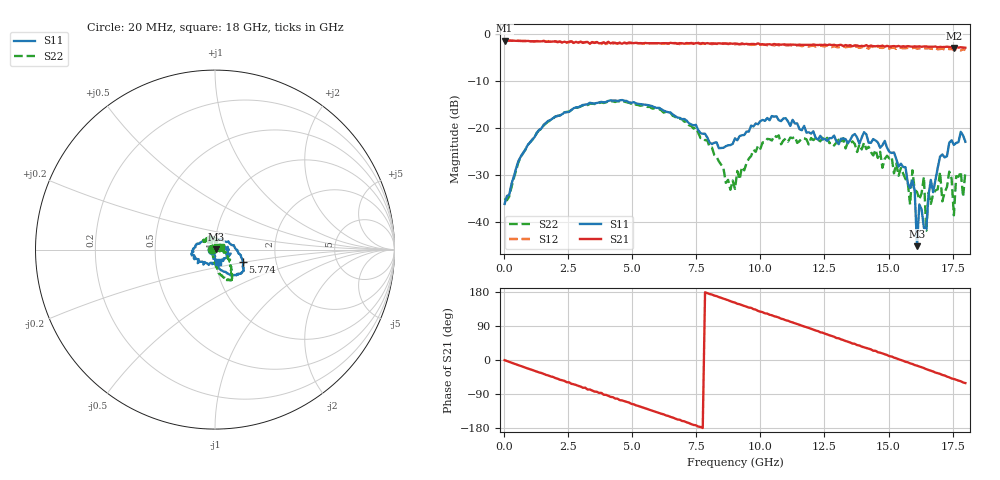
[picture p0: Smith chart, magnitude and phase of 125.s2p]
!Agilent Technologies,N5230A,US43500223,A.07.50.48
!Agilent N5230A: A.07.50.48
!Date: Tuesday, February 02, 2016 14:28:02
!Correction: S11(Full 2 Port(1,2))
!S21(Full 2 Port(1,2))
!S12(Full 2 Port(1,2))
!S22(Full 2 Port(1,2))
!S2P File: Measurements: S11, S21, S12, S22:
# Hz S  RI  R 50
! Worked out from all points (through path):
!   201 points, 20 MHz to 18 GHz, reference 50 ohm
!   highest |S21| = -1.32 dB at 20 MHz (marker M1); lowest = -2.9 dB at 17.55 GHz (marker M2)
!   group delay of S21, straight-line fit = 64.6 ps
!   lowest |S11| = -45.2 dB at 16.11 GHz (marker M3), VSWR 1.01, Z = 50.5 + j0.115 ohm
!   |S11| at or under -10 dB: start of sweep to end of sweep
!   |S22| runs from -41.9 to -14.3 dB; largest |S21 - S12| = 0.11
!   S11 on the Smith chart (normalised r, x): 20 MHz: 0.97, +0.00; 5.774 GHz: 1.36, -0.19; 18 GHz: 1.02, -0.14
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2e7  -0.0155 0.000255  0.8591 -0.00723  0.86 -0.0116  -0.0179 0.000888
1.2786e9  0.0115 -0.0887  0.7254 -0.4307  0.7272 -0.4344  0.00456 -0.0884
3.0766e9  0.103 -0.1431  0.2321 -0.7755  0.2216 -0.7891  0.0598 -0.1632
5.7736e9  0.1567 -0.0693  -0.5531 -0.584  -0.5767 -0.5584  0.0906 -0.1339
6.0433e9  0.155 -0.0555  -0.6129 -0.5207  -0.6336 -0.4911  0.0975 -0.1272
9.01e9  -0.0468 0.062  -0.7008 0.3827  -0.662 0.4162  0.00671 0.0214
1.02686e10  -0.1278 -0.00772  -0.4196 0.6598  -0.3502 0.6799  -0.062 0.0451
1.20666e10  -0.0351 -0.0852  0.1308 0.7681  0.1996 0.7354  -0.0365 0.0648
1.50333e10  0.0513 0.0218  0.7296 0.1297  0.7034 0.0536  -0.00156 0.0473
1.58424e10  0.00251 0.0228  0.7334 -0.1139  0.6833 -0.1878  -0.00134 0.0152
1.59323e10  0.012 0.0249  0.7256 -0.1336  0.6813 -0.2041  0.014 0.0325
1.61121e10  0.00538 0.00113  0.715 -0.1914  0.6533 -0.261  -0.00147 0.0208
1.6202e10  -0.0149 0.00336  0.7127 -0.2191  0.649 -0.2827  0.0107 0.0136
1.63818e10  0.00861 0.000151  0.6914 -0.2684  0.6226 -0.3435  0.028 0.0109
1.64717e10  0.0042 -0.00717  0.6784 -0.3048  0.6111 -0.3573  0.00713 0.00366
1.65616e10  -0.00609 -0.0181  0.6605 -0.325  0.5964 -0.3855  0.0124 0.0163
1.7101e10  -0.00866 -0.0516  0.5638 -0.4654  0.4828 -0.5115  0.0139 -0.00887
1.73707e10  0.0139 -0.0684  0.5107 -0.5246  0.4158 -0.5586  0.0333 0.00804
1.75505e10  0.00836 -0.0656  0.4594 -0.5488  0.3651 -0.5754  0.00979 0.00643
1.76404e10  0.0144 -0.0678  0.4501 -0.5783  0.3622 -0.592  0.0304 0.00384
1.79101e10  0.0195 -0.081  0.3693 -0.6218  0.2851 -0.6344  0.0184 -0.00111
1.8e10  0.0161 -0.0696  0.3502 -0.6292  0.2451 -0.6338  0.0322 0.0128
